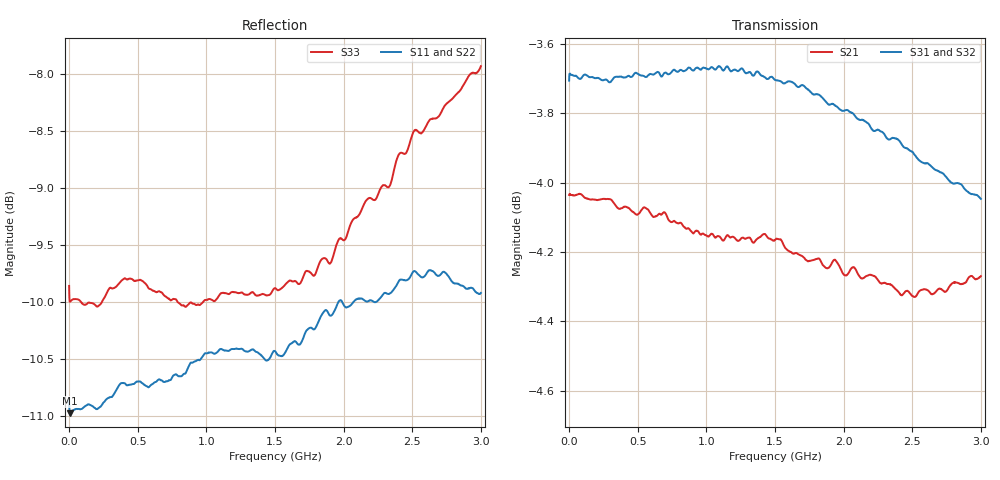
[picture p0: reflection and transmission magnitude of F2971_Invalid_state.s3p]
! Frequency:  300kHz to 3GHz
! Package:  4mm x 4mm LQFN Plastic Package: 20 pin with exposed paddle.
!  Pin 1,2,4,5,6,7,9,10,11,12,14,15,18,19 = GND
!  Pin 3  = RF1  = Port 1
!  Pin 8  = RFC  = Port 3
!  Pin 13 = RF2  = Port 2
!  Pin 16 = C2
!  Pin 17 = C1
!  Pin 20 = VDD
!  E.P.  = GND
! State:  Invalid State
! Voltage:  VDD  = +3.0V
!  C1  = +3.0V (Logic HIGH)
!  C2  = +3.0V (Logic HIGH)
! Data:  The device was measured on the F2971 EVKit using a calibrated
!  network analyzer. The results below remove the PCB trace and
!  connector effects using the Automatic Fixture Removal software
!  from Keysight. Therfore, the reference plane for these results
!  are at the device's RF pin.
! Misc:
! Date:  2018-03-27  SJ
! Note:
!  Integrated Device Technology supplies this data as a sample of
!  measured data. Data was taken at 25 degrees C. Integrated Device
!  Technology reserves the right to change this data at anytime.
# hz S db R 75
! 3 Port Network Data from SP1.SP block
! freq  dbS11  angS11  dbS12  angS12  dbS13  angS13
!  dbS21  angS21
!  dbS22  angS22  dbS23  angS23
!  dbS31  angS31  dbS32  angS32
!  dbS33  angS33
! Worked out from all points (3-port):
!   1601 points, 30 kHz to 3 GHz, reference 75 ohm
!   strongest paths, dB at 30 kHz, 750 MHz, 1.5 GHz, 2.25 GHz, 3 GHz:
!     S31: -3.7, -3.7, -3.7, -3.8, -4.0
!     S32: -3.7, -3.7, -3.7, -3.9, -4.1
!     S21: -4.0, -4.1, -4.2, -4.3, -4.3
!   lowest |S11| = -11.0 dB at 7.53 MHz (marker M1), VSWR 1.79, Z = 41.9 + j0.0749 ohm
!   |S11| at or under -10 dB: start of sweep to 1.96 GHz; 1.992 GHz to 2.069 GHz (77.46 MHz wide, 3.81 % of centre)
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30000  -10.84 177.5  -4.03 0.1  -3.70 0.3
       -4.04 0.1  -10.84 177.5  -3.70 0.2
       -3.71 0.3  -3.70 0.3  -9.85 177.6
7529925  -10.97 179.8  -4.04 -0.2  -3.69 -0.2
         -4.03 -0.2  -10.97 179.9  -3.68 -0.2
         -3.69 -0.1  -3.68 -0.1  -9.99 179.9
7.687723e8  -10.63 170.8  -4.11 -16.2  -3.67 -14.3
            -4.11 -16.1  -10.69 171.5  -3.68 -14.3
            -3.68 -14.3  -3.68 -14.3  -9.97 175.1
1.096894e9  -10.41 168.6  -4.16 -22.9  -3.66 -20.8
            -4.16 -22.9  -10.40 168.8  -3.68 -20.5
            -3.66 -20.8  -3.68 -20.6  -9.93 172.6
1.500015e9  -10.43 167.5  -4.17 -31.1  -3.70 -28.6
            -4.17 -31.1  -10.52 167.4  -3.71 -28.3
            -3.70 -28.7  -3.71 -28.3  -9.87 171.8
1.905011e9  -10.12 166.6  -4.24 -39.6  -3.78 -36.6
            -4.24 -39.5  -10.12 166.3  -3.79 -36.1
            -3.77 -36.6  -3.79 -36.1  -9.65 170.1
2.555629e9  -9.77 163.3  -4.31 -52.7  -3.94 -49.0
            -4.31 -52.6  -9.62 162.8  -3.97 -48.3
            -3.94 -49.0  -3.97 -48.3  -8.51 166.0
2.746878e9  -9.75 161.1  -4.32 -56.3  -3.98 -52.6
            -4.31 -56.2  -9.43 160.8  -4.03 -51.7
            -3.98 -52.6  -4.03 -51.7  -8.26 162.9
2.925001e9  -9.87 157.7  -4.27 -59.7  -4.03 -55.9
            -4.27 -59.6  -9.78 158.3  -4.05 -54.9
            -4.03 -55.9  -4.05 -55.0  -8.00 160.0
3e9  -9.92 155.6  -4.27 -61.2  -4.04 -57.2
     -4.27 -61.1  -9.64 156.6  -4.07 -56.1
     -4.05 -57.2  -4.07 -56.2  -7.93 158.3
